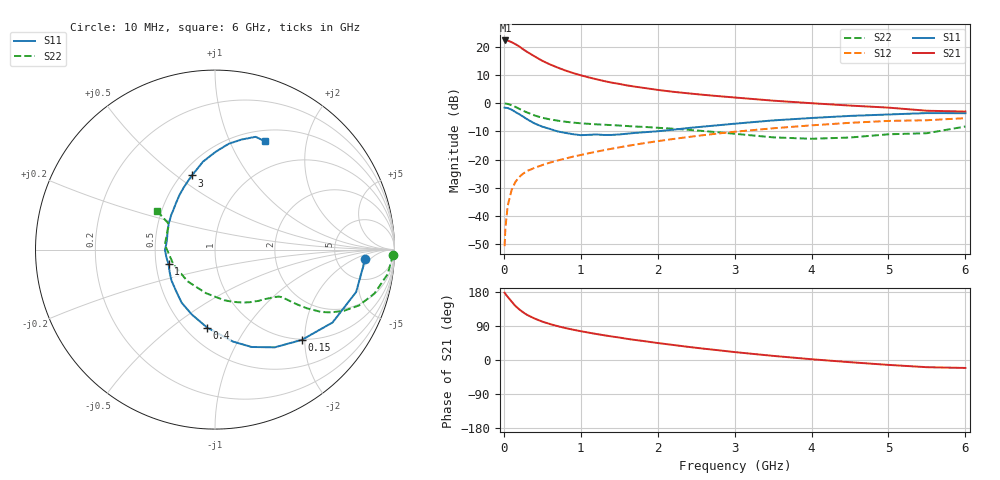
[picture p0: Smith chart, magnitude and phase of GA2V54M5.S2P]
! Infineon Technologies  Discrete & RF Semiconductors
! BF775
! Si NPN RF Bipolar Junction Transistor in SOT23
! VCE = 2.5 V  IC = 4.5 mA
! Common Emitter S-Parameters:  May  1996
# GHz  S  MA  R  50
!  f  S11  S21  S12  S22
! GHz  MAG  ANG  MAG  ANG  MAG  ANG  MAG  ANG
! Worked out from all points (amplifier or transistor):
!   36 points, 10 MHz to 6 GHz, reference 50 ohm
!   highest |S21| = 22.3 dB at 20 MHz (marker M1)
!   |S21| within 3 dB of that: start of sweep to 244.1 MHz
!   unconditionally stable (mu >= 1): 818.9 MHz to 3.745 GHz
!   at 250 MHz: K = 0.46, MSG = 22.1 dB, |S12| = -25.0 dB
!   at 1.4 GHz: K = 1.14, MAG = 9.5 dB, |S12| = -16.2 dB
!   at 6 GHz: K = 0.98, MSG = 1.2 dB, |S12| = -5.3 dB
!   S11 on the Smith chart (normalised r, x): 10 MHz: 10, -3; 150 MHz: 0.99, -1.94; 400 MHz: 0.63, -0.68; 1 GHz: 0.58, -0.10; 3 GHz: 0.56, +0.57; 6 GHz: 0.63, +1.36
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0.01  0.8355 -3.5  12.98 177.5  0.0029 88.2  0.9922 -1.6
0.02  0.8306 -6.7  13 174.4  0.006 84.6  0.9861 -3.2
0.05  0.8212 -16.7  12.96 166.6  0.0151 81.4  0.9715 -8.1
0.1  0.7706 -31.8  12.14 154.5  0.0285 73.9  0.9214 -15.4
0.15  0.6979 -46.1  11.18 142.6  0.0401 67.1  0.8605 -21.2
0.2  0.6381 -58.6  10.18 133.7  0.049 62.7  0.7949 -25.4
0.25  0.5797 -69.4  9.079 125.9  0.0561 58.8  0.7355 -28.4
0.3  0.5218 -79.0  8.185 119.3  0.0625 57.1  0.6872 -30.4
0.4  0.437 -95.7  6.779 109.4  0.0712 54.3  0.606 -32.6
0.5  0.3836 -109.8  5.654 101.3  0.0798 53.9  0.5511 -33.7
0.6  0.3492 -122.2  4.882 94.9  0.0883 53.7  0.5165 -34.3
0.8  0.2973 -144.7  3.807 84.3  0.1041 53.9  0.4693 -35.2
1  0.271 -162.9  3.131 76.0  0.1204 55.0  0.4404 -36.5
1.1  0.2743 -170.8  2.881 72.3  0.1292 55.1  0.4311 -37.7
1.3  0.2733 173.6  2.481 65.4  0.1466 54.9  0.4151 -39.9
1.6  0.2875 156.1  2.071 55.9  0.1739 54.3  0.3939 -44.3
2.2  0.3379 130.1  1.596 39.7  0.2316 50.8  0.3528 -56.1
3  0.4328 107.2  1.263 20.9  0.3115 43.2  0.2868 -79.7
3.5  0.495 97.7  1.11 10.9  0.3588 37.1  0.2477 -101.9
4.5  0.5952 82.5  0.908 -5.8  0.4487 24.2  0.246 -160.3
5.5  0.6679 70.2  0.735 -19.0  0.4985 9.3  0.2934 151.0
6  0.6648 65.2  0.711 -21.0  0.543 5.2  0.3859 146.4
